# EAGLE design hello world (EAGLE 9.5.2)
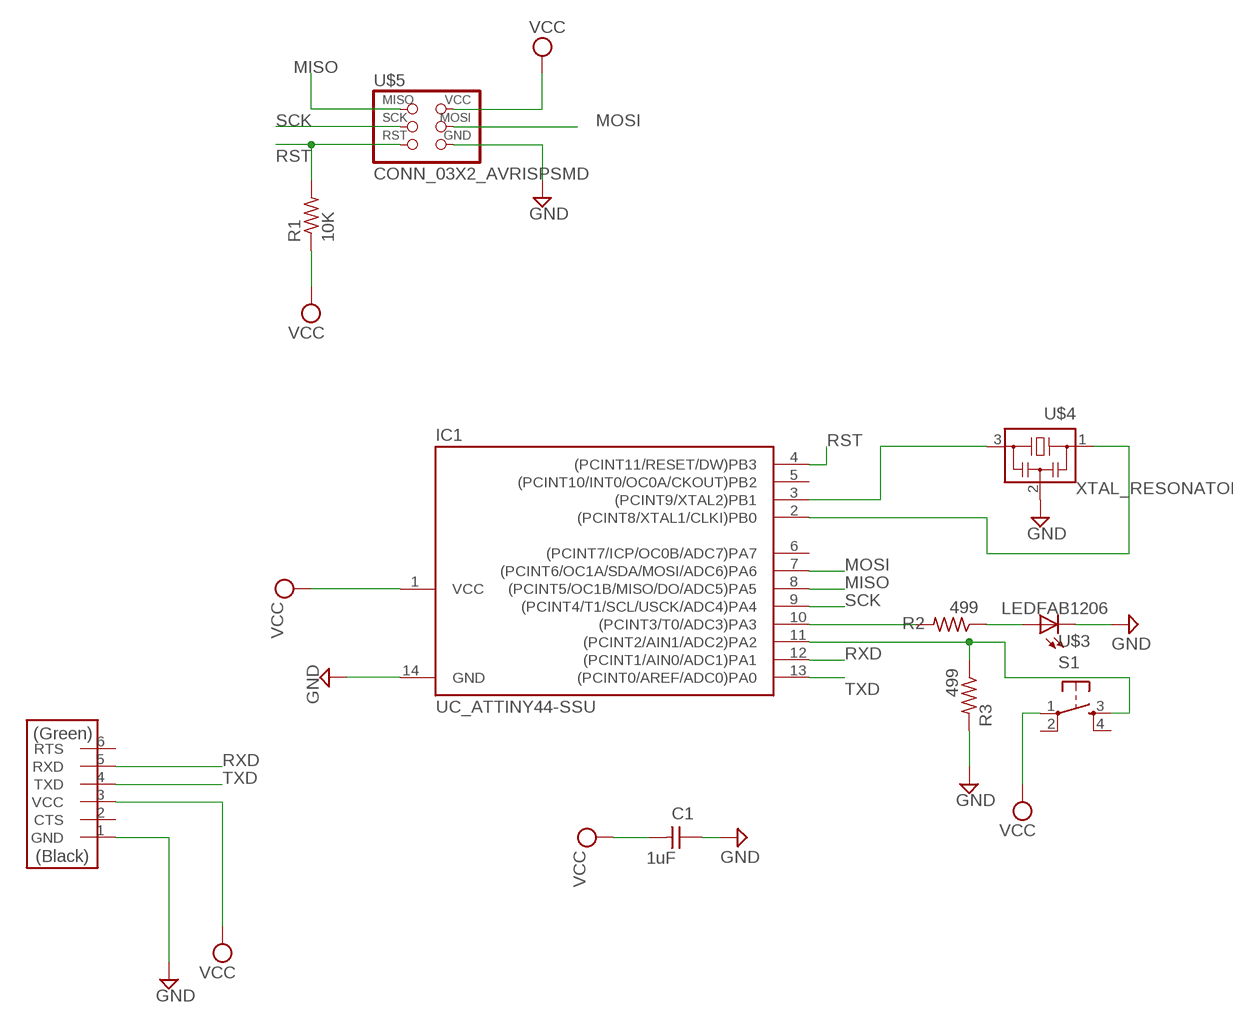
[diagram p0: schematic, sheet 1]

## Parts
C1  1uF  CAP_UNPOLARIZEDFAB  [C1206FAB]
IC1  UC_ATTINY44-SSU  [SOIC14]
R1  10K  R1206  [R1206]
R2  499  R1206  [R1206]
R3  499  R1206  [R1206]
S1  SW_SWITCH_TACTILE_6MM6MM_SWITCH  [6MM_SWITCH]
U$1  CONN_06_FTDI-SMD-HEADER  [1X06SMD]
U$3  LEDFAB1206  [LED1206FAB]
U$4  XTAL_RESONATOR  [EFOBM]
U$5  CONN_03X2_AVRISPSMD  [2X03SMD]

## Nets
GND: C1.1 IC1.14(GND) R3.2 U$1.1(GND) U$3.2(C) U$4.2 U$5.6(GND)
MISO: IC1.8((PCINT5/OC1B/MISO/DO/ADC5)PA5) U$5.1(MISO)
MOSI: IC1.7((PCINT6/OC1A/SDA/MOSI/ADC6)PA6) U$5.4(MOSI)
N$1: IC1.10((PCINT3/T0/ADC3)PA3) R2.2
N$2: R2.1 U$3.1(A)
N$3: IC1.11((PCINT2/AIN1/ADC2)PA2) R3.1 S1.3(S)
N$5: IC1.3((PCINT9/XTAL2)PB1) U$4.3
N$6: IC1.2((PCINT8/XTAL1/CLKI)PB0) U$4.1
RST: IC1.4((PCINT11/RESET/DW)PB3) R1.2 U$5.5(RST)
RXD: IC1.12((PCINT1/AIN0/ADC1)PA1) U$1.5(RXD)
SCK: IC1.9((PCINT4/T1/SCL/USCK/ADC4)PA4) U$5.3(SCK)
TXD: IC1.13((PCINT0/AREF/ADC0)PA0) U$1.4(TXD)
VCC: C1.2 IC1.1(VCC) R1.1 S1.1(P) U$1.3(VCC) U$5.2(VCC)
Unconnected: IC1.5((PCINT10/INT0/OC0A/CKOUT)PB2) IC1.6((PCINT7/ICP/OC0B/ADC7)PA7) S1.2(P1) S1.4(S1) U$1.2(CTS) U$1.6(RTS)

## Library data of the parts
C1 = fab:CAP_UNPOLARIZED
IC1 = fab:UC_ATTINY44
R1-R3 = fab:R: Resistor (US Symbol)
S1 = fab:SW_SWITCH_TACTILE_6MM: OMRON SWITCH
U$1 = fab:CONN_06_FTDI-SMD-HEADER
U$3 = fab:LED: LED
U$4 = fab:XTAL_RESONATOR
U$5 = fab:CONN_03X2_AVRISP

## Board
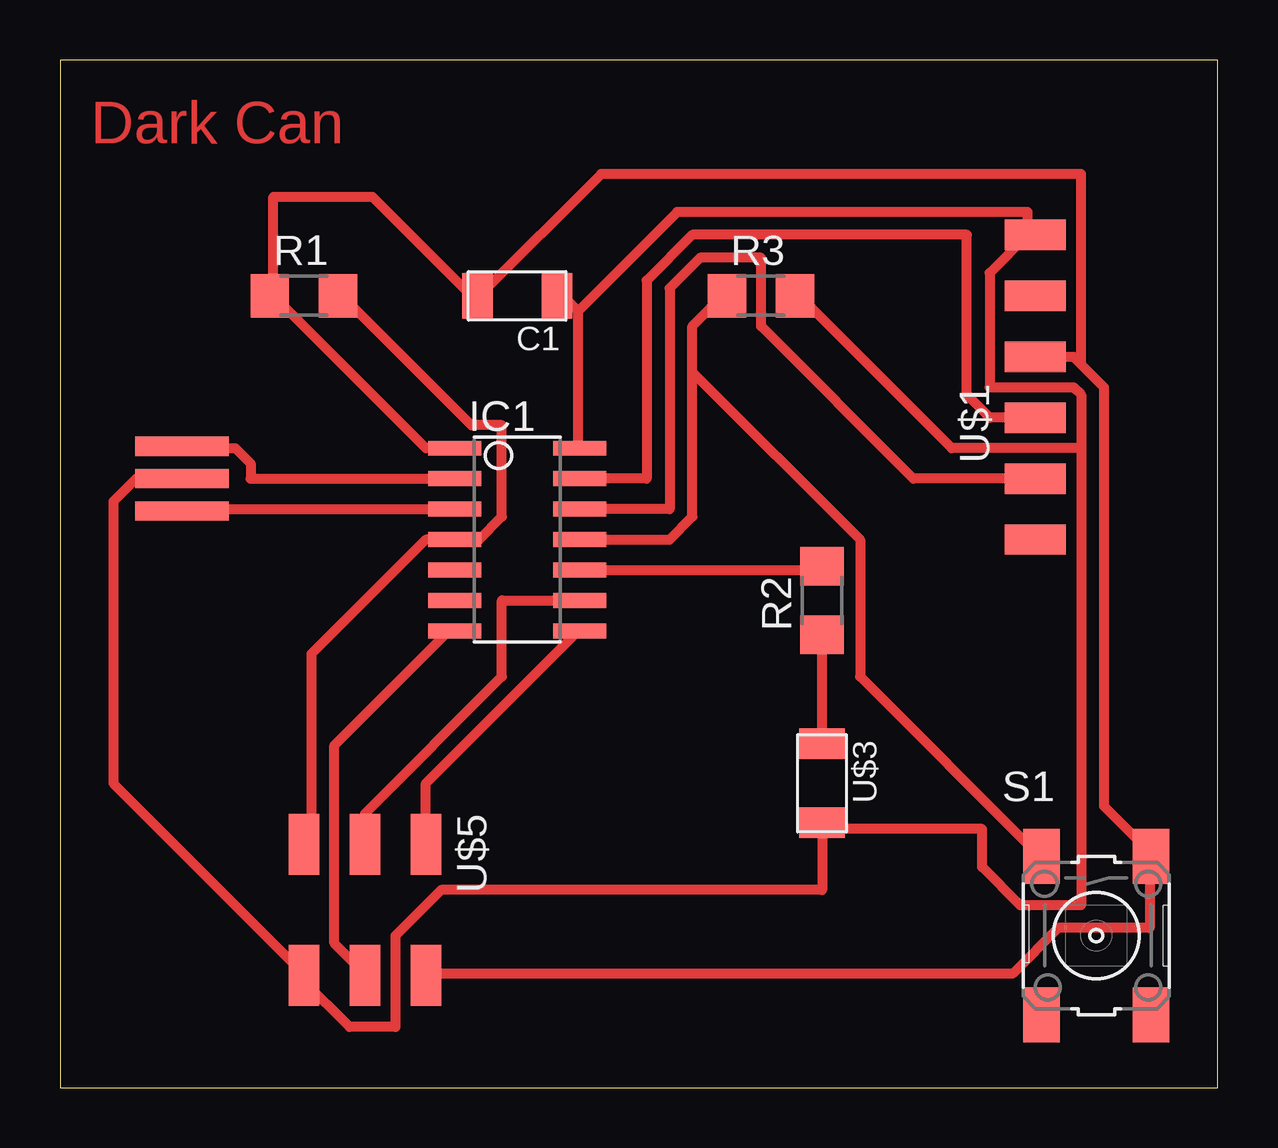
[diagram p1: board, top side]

Size 48.24 x 42.85 mm. Coordinates in mm from the lower left corner, seen from the top.
Outline: 0,0 48.24,0 48.24,42.85 0,42.85 0,0
Copper layers (1*16): Top 0.035mm / dielectric 1.5mm / Bottom 0.035mm
Design rules "fab *": minimum track width 16mil, minimum drill 32mil, track to track 16mil, track to pad 16mil, pad to pad 16mil, via to via 16mil, smd to smd 6mil, copper to edge 16mil, drill to drill 16mil, minimum pad ring 10mil, minimum via ring 8mil, stop-mask expansion 4mil, vias tented up to drill 0mil, thermal gap 16mil

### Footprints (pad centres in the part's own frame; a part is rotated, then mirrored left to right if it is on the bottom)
C1206FAB = smd 1.27 x 1.905: 1 -1.651,0; 2 1.651,0
SOIC14 = smd 0.61 x 2.21: 1 -3.81,-2.603; 2 -2.54,-2.603; 3 -1.27,-2.603; 4 0,-2.603; 5 1.27,-2.603; 6 2.54,-2.603; 7 3.81,-2.603; 8 3.81,2.603; 9 2.54,2.603; 10 1.27,2.603; 11 0,2.603; 12 -1.27,2.603; 13 -2.54,2.603; 14 -3.81,2.603
R1206 = smd 1.6 x 1.803: 1 -1.422,0; 2 1.422,0
6MM_SWITCH = smd 2.286 x 1.524: 1 -3.302,2.286; 2 3.302,2.286; 3 -3.302,-2.286; 4 3.302,-2.286
1X06SMD = smd 2.54 x 1.27: 1 0,6.35; 2 0,3.81; 3 0,1.27; 4 0,-1.27; 5 0,-3.81; 6 0,-6.35
LED1206FAB = smd 1.27 x 1.905: 1 -1.651,0; 2 1.651,0
EFOBM = smd 0.8 x 3.9: 1 -1.35,0; 2 0,0; 3 1.35,0
2X03SMD = smd 2.54 x 1.27: 1 -2.54,2.54; 2 2.92,2.54; 3 -2.54,0; 4 2.92,0; 5 -2.54,-2.54; 6 2.92,-2.54

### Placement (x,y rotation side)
C1  19.05,33.02 180 top
IC1  19.05,22.86 270 top
R1  10.16,33.02 0 top
R2  31.75,20.32 90 top
R3  29.21,33.02 0 top
S1  43.18,6.35 270 top
U$1  40.64,29.21 0 top
U$3  31.75,12.7 270 top
U$4  5.08,25.4 270 top
U$5  12.7,7.62 270 top

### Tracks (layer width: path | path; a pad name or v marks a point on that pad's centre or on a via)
GND
  Top 0.406: U$4.2 3.17,25.4 2.22,24.45 2.22,12.7 10.16,4.76 U$5.6 10.16,4.45 12.06,2.54 13.97,2.54 13.97,6.35 15.88,8.26 31.75,8.26 31.75,10.79 | 21.59,32.38 20.95,33.02 C1.1 | 21.59,32.38 21.59,26.67 IC1.14 | 42.55,26.67 37.15,26.67 30.8,33.02 R3.2 | 42.55,26.67 42.55,28.89 42.23,29.21 38.73,29.21 38.73,33.97 40.32,35.56 | 31.75,10.79 38.42,10.79 38.42,9.21 40.01,7.62 42.55,7.62 42.55,26.67 | 21.59,32.38 25.72,36.51 40.32,36.51 40.32,35.56 | 40.32,35.56 U$1.1 | 31.75,10.79 U$3.2
MISO
  Top 0.406: U$5.1 15.24,12.7 21.59,19.05 IC1.8
MOSI
  Top 0.406: IC1.7 16.19,19.05 11.43,14.29 11.43,6.03 12.7,4.76 U$5.4
N$1
  Top 0.406: IC1.10 31.75,21.59 R2.2
N$2
  Top 0.406: U$3.1 R2.1
N$3
  Top 0.406: 26.35,29.84 26.35,23.81 25.4,22.86 IC1.11 | 26.35,29.84 26.35,31.75 27.62,33.02 R3.1 | 26.35,29.84 33.34,22.86 33.34,17.14 40.64,9.84 S1.3
N$5
  Top 0.406: IC1.3 5.08,24.13 U$4.3
N$6
  Top 0.406: IC1.2 7.94,25.4 7.94,26.04 7.3,26.67 5.08,26.67 U$4.1
RST
  Top 0.406: R1.2 11.75,33.02 17.14,27.62 18.41,27.62 18.41,23.81 17.46,22.86 IC1.4 15.24,22.86 10.48,18.1 10.48,10.48 U$5.5
RXD
  Top 0.406: IC1.12 25.4,24.13 25.4,33.34 26.67,34.61 29.21,34.61 29.21,31.75 35.56,25.4 U$1.5
SCK
  Top 0.406: IC1.9 18.41,20.32 18.41,17.14 12.7,11.43 U$5.3
TXD
  Top 0.406: IC1.13 24.45,25.4 24.45,33.66 26.35,35.56 37.78,35.56 37.78,28.89 38.73,27.94 U$1.4
VCC
  Top 0.406: 8.89,33.02 15.24,26.67 IC1.1 | 8.89,33.02 8.89,37.15 13.02,37.15 17.14,33.02 C1.2 17.46,33.02 22.54,38.1 42.55,38.1 42.55,30.16 | 8.89,33.02 R1.1 | 42.55,30.16 42.23,30.48 U$1.3 | 42.55,30.16 43.5,29.21 43.5,11.75 45.4,9.84 S1.1 45.4,9.53 45.4,6.67 41.59,6.67 39.69,4.76 15.24,4.76 U$5.2

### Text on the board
Top: Dark Can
